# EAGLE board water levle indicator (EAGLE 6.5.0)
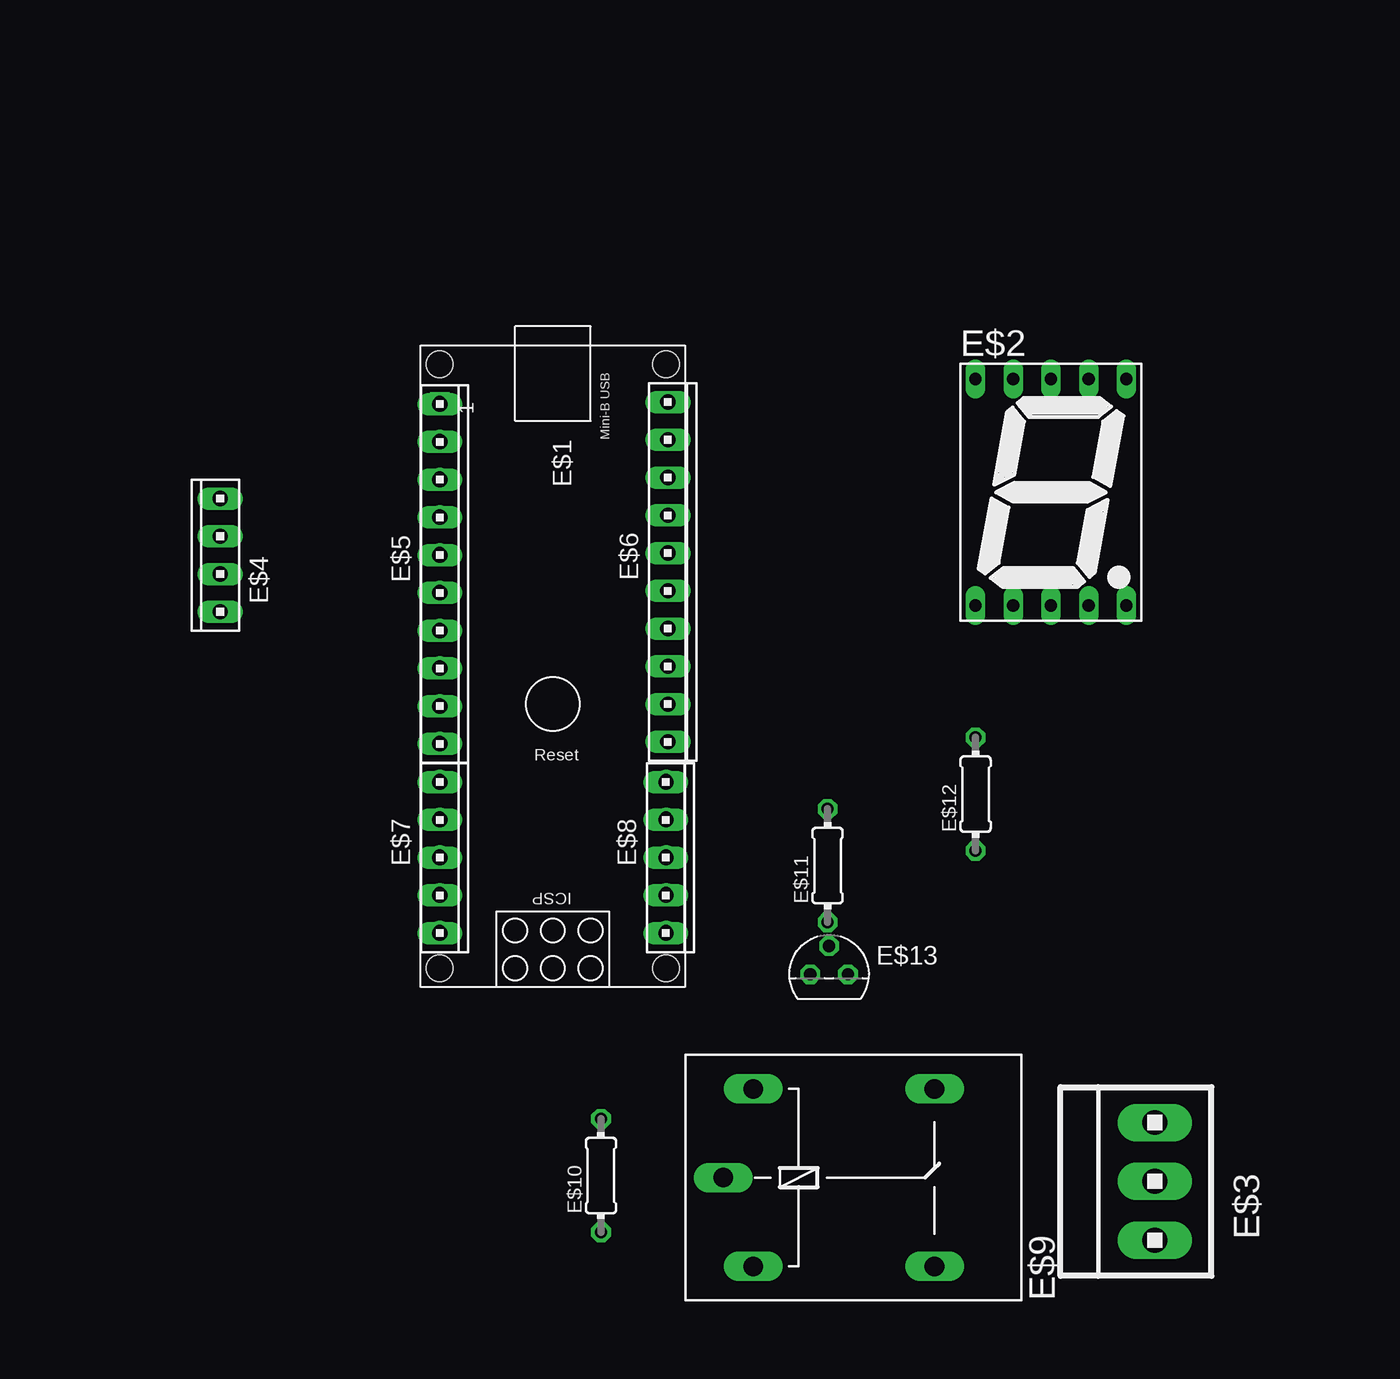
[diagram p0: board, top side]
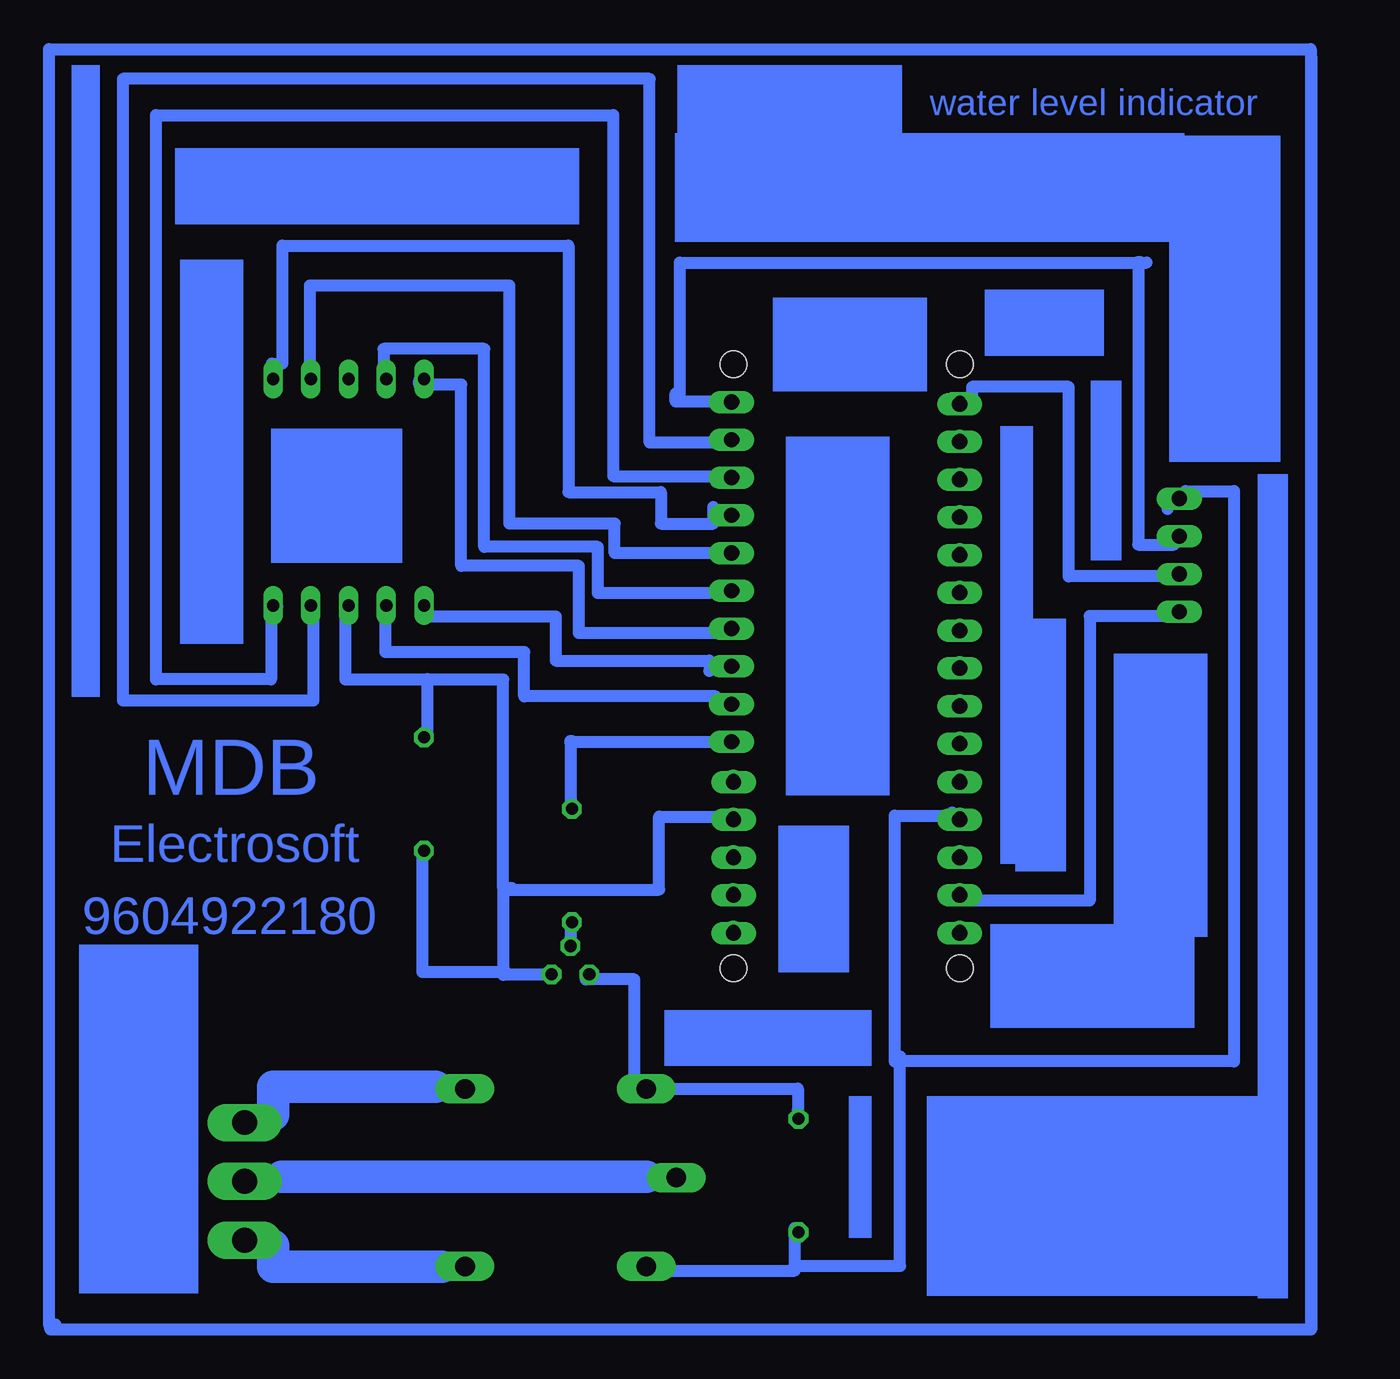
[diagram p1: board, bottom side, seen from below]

No outline drawn. Coordinates in mm, seen from the top.
Copper layers (1*16): Top 0.035mm / dielectric 1.5mm / Bottom 0.035mm
Design rules "default": minimum track width 10mil, minimum drill 24mil, track to track 8mil, track to pad 8mil, pad to pad 8mil, via to via 8mil, smd to smd 8mil, copper to edge 40mil, drill to drill 8mil, minimum pad ring 10mil, minimum via ring 8mil, stop-mask expansion 4mil, vias tented up to drill 0mil, thermal gap 10mil

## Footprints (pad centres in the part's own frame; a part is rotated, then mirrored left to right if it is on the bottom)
ARDUINO_NANO = drill 0.8 square: 1 -20.32,-7.62 | drill 0.8: 2 -17.78,-7.62; 3 -15.24,-7.62; 4 -12.7,-7.62; 5 -10.16,-7.62; 6 -7.62,-7.62; 7 -5.08,-7.62; 8 -2.54,-7.62; 9 0,-7.62; 10 2.54,-7.62; 11 5.08,-7.62; 12 7.62,-7.62; 13 10.16,-7.62; 14 12.7,-7.62; 15 15.24,-7.62; 16 15.24,7.62; 17 12.7,7.62; 18 10.16,7.62; 19 7.62,7.62; 20 5.08,7.62; 21 2.54,7.62; 22 0,7.62; 23 -2.54,7.62; 24 -5.08,7.62; 25 -7.62,7.62; 26 -10.16,7.62; 27 -12.7,7.62; 28 -15.24,7.62; 29 -17.78,7.62; 30 -20.32,7.62 | hole 1.778: -22.86,-7.62; -22.86,7.62; 17.78,7.62; 17.78,-7.62
7SEG-13 = drill 0.813 long: 1 -5.08,-7.62; 2 -2.54,-7.62; 3 0,-7.62; 4 2.54,-7.62; 5 5.08,-7.62; 6 5.08,7.62; 7 2.54,7.62; 8 0,7.62; 9 -2.54,7.62; 10 -5.08,7.62
1X3MTA = drill 1.676 long: 1 3.937,0; 2 -0.025,0; 3 -3.988,0
10X04MTA = drill 1.016 long: 1 3.81,0; 2 1.27,0; 3 -1.27,0; 4 -3.81,0
10X10MTA = drill 1.016 long: 1 11.43,0; 2 8.89,0; 3 6.35,0; 4 3.81,0; 5 1.27,0; 6 -1.27,0; 7 -3.81,0; 8 -6.35,0; 9 -8.89,0; 10 -11.43,0
10X05MTA = drill 1.016 long: 1 5.08,0; 2 2.54,0; 3 0,0; 4 -2.54,0; 5 -5.08,0
G5LE = drill 1.321 long: 1 -7.493,-5.969; 2 -7.493,5.969; O 4.699,5.969; P -9.525,0; S 4.699,-5.969
0204/7 = drill 0.813 octagon: 1 -3.81,0; 2 3.81,0
TO92 = drill 0.813 octagon: 1 1.27,0; 2 0,1.905; 3 -1.27,0

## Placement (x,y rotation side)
E$1  [ARDUINO_NANO]  39.71,45.26 270 top
E$2  [7SEG-13]  73.23,59.51 0 top
E$3  [1X3MTA]  80.23,13.17 90 top
E$4  [10X04MTA]  17.32,55.28 90 top
E$5  [10X10MTA]  32.11,54.01 270 top
E$6  [10X10MTA]  47.46,54.15 270 top
E$7  [10X05MTA]  32.11,34.92 270 top
E$8  [10X05MTA]  47.32,34.92 270 top
E$9  [G5LE]  60.7,13.4 0 top
E$10  [0204/7]  42.95,13.54 90 top
E$11  [0204/7]  58.2,34.39 90 top
E$12  [0204/7]  68.16,39.2 90 top
E$13  [TO92]  58.3,27.07 0 top

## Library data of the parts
E$1 = ArduinoNanoV30 (1)
E$2 = special
E$3-E$8 = con-amp
E$9 = relay
E$10-E$12 = resistor
E$13 = transistor

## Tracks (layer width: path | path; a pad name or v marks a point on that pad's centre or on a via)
S$1
  Bottom 0.813: 48.25,65.6 51.22,65.6 51.22,66.17 50.94,66.17 50.94,74.95 19.53,74.95
S$2
  Bottom 0.813: 18.39,53.84 24.76,53.84 24.76,66.59 31.27,66.59 31.27,65.17
S$3
  Bottom 0.813: 16.91,59.58 13.65,59.58 13.65,21.22 36.47,21.22 36.47,37.74 32.6,37.74 32.6,37.95
S$4
  Bottom 0.813: 48.49,62.84 52.98,62.84 52.98,87.32 88.43,87.32 88.43,45.5 75.59,45.5 75.59,51.01
S$5
  Bottom 0.813: 78.04,51.82 78.45,51.82 78.45,46.92 86.19,46.92 86.19,84.87 55.42,84.87 55.42,60.59 48.49,60.59 48.49,60.19
S$6
  Bottom 2.184: 67.39,19.52 78.29,19.52 78.29,17.64
S$7
  Bottom 2.184: 53.19,13.45 77.74,13.45
S$8
  Bottom 2.184: 66.95,7.39 78.29,7.39 78.29,8.82
S$9
  Bottom 0.813: 52.16,7.14 43.2,7.14 43.2,10
S$10
  Bottom 0.813: 52.57,19.38 42.99,19.38 42.99,17.95
S$11
  Bottom 0.813: 54,18.97 54,26.73 57.26,26.73 57.26,26.93
S$12
  Bottom 0.813: 59.86,27.04 62.81,27.04 62.81,32.77 52.33,32.77 52.33,37.69 48.4,37.69
S$13
  Bottom 0.813: 43.24,7.46 36.11,7.46 36.11,21.55
S$14
  Bottom 0.813: 48.23,42.68 58.31,42.68
S$15
  Bottom 0.813: 58.23,42.76 58.31,42.76 58.31,38.42
S$16
  Bottom 0.813: 58.14,30.31 58.31,30.31 58.31,29.49
S$17
  Bottom 0.813: 62.26,32.88 62.83,32.88 62.83,46.91 73.44,46.91 73.44,51.44
S$18
  Bottom 0.813: 48.53,45.77 61.41,45.77 61.41,48.75 70.75,48.75 70.75,51.72
S$19
  Bottom 0.813: 67.92,51.16 59.29,51.16 59.29,48.18 48.96,48.18 48.96,47.47
S$20
  Bottom 0.813: 48.39,50.02 57.73,50.02 57.73,54.56 65.66,54.56 65.66,66.75 68.49,66.75 68.49,67.03
S$21
  Bottom 0.813: 48.96,52.72 56.46,52.72 56.46,55.83 64.1,55.83 64.1,69.15 70.89,69.15 70.89,67.59
S$22
  Bottom 0.813: 48.96,55.41 55.33,55.41 55.33,57.39 62.4,57.39 62.4,73.41 75.84,73.41 75.84,67.59
S$23
  Bottom 0.813: 78.39,68.16 77.68,68.16 77.68,76.1 58.44,76.1 58.44,59.52 52.21,59.52 52.21,57.39 48.68,57.39 48.68,58.53
S$24
  Bottom 0.813: 18.25,51.17 23.35,51.17 23.35,32.03 31.41,32.03 31.41,32.74
S$25
  Bottom 0.813: 18.11,58.94 18.11,58.37
S$26
  Bottom 0.813: 19.95,74.98 20.09,74.98 20.09,55.99 17.69,55.99
S$27
  Bottom 0.813: 62.66,27.22 68.26,27.22 68.26,35.38
S$28
  Bottom 0.813: 68.26,43.21 67.92,43.21 67.92,46.95
S$29
  Bottom 0.813: 8.45,88.84 8.45,3.17 93.31,3.17 93.31,3.53 92.95,3.53
S$31
  Bottom 0.813: 93.38,3.53 93.38,89.31 8.48,89.31 8.48,3.2
(copper drawn outside any net)
  shapes: Bottom area x21

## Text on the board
Bottom: water level indicator | MDB | Electrosoft | 9604922180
